DATA_BLOCK "MGUD"
TITLE =
VERSION : 0.1


  STRUCT
   ALB_BUFFER : INT ;
   VASS_BUFFER : INT ;
   ALB_GREZZI : INT ;
   VASS_GREZZI : INT ;
   ALB_FINITI : INT ;
   VASS_FINITI : INT ;
   ORIG_ALB_PP : INT ;
   ORIG_ALB_BSX_P1 : INT ;
   ORIG_ALB_BSX_P2 : INT ;
   ORIG_ALB_BDX_P1 : INT ;
   ORIG_ALB_BDX_P2 : INT ;
   ZN_CEN_PRE_BSX : INT ;
   ZN_CEN_OCC_BSX : INT ;
   ZN_CEN_PRE_BDX : INT ;
   ZN_CEN_OCC_BDX : INT ;
   ALB_ESTRATTI : INT ;
   VAR_DISP : INT ;
   VAR_DISP1 : INT ;
   VAR_DISP2 : INT ;
   VAR_DISP3 : INT ;
   VAR_DISP4 : INT ;
   VAR_DISP5 : INT ;
   VAR_DISP6 : INT ;
   VAR_DISP7 : INT ;
   VAR_DISP8 : INT ;
      Y_SX_ATTESA_MSX : REAL ;
   Y_SX_DISCESA_MSX : REAL ;
   Z_SX_ALTO : REAL ;
   Z_SX_PREL_MSX : REAL ;
   Z_SX_DEP_MSX : REAL ;
   Z_SX_SVINC_MSX : REAL ;
   C_SX_PREL_MSX : REAL ;
   A_SX_PREL_MSX : REAL ;
   A_SX_DEP_MSX : REAL ;
   MSX_DISP1 : REAL ;
   MSX_DISP2 : REAL ;
   MSX_DISP3 : REAL ;
   MSX_DISP4 : REAL ;
   MSX_DISP5 : REAL ;
   MSX_DISP6 : REAL ;
   MSX_DISP7 : REAL ;
   MSX_DISP8 : REAL ;
   Y_SX_DISCESA_PP : REAL ;
   Z_SX_ALTO_PP : REAL ;
   Z_SX_PREL_PP : REAL ;
   Z_SX_SVINC_PP : REAL ;
   C_SX_PREL_PP : REAL ;
   A_SX_PREL_PP : REAL ;
   A_SX_DEP_PP : REAL ;
   PP_DISP1 : REAL ;
   PP_DISP2 : REAL ;
   PP_DISP3 : REAL ;
   PP_DISP4 : REAL ;
   PP_DISP5 : REAL ;
   PP_DISP6 : REAL ;
   PP_DISP7 : REAL ;
   PP_DISP8 : REAL ;
   Z_SX_SVINC_PALLET : REAL ;
   Z_SX_PREL_PALLET : REAL ;
   Z_SX_DEP_PALLET : REAL ;
   Z_SX_PREL_ALBERI : REAL ;
   Y_SX_PREL_PALLET : REAL ;
   Y_SX_DEP_PALLET : REAL ;
   Y_SX_PREL_ALBERI : REAL ;
   A_SX_PREL_GREZZI : REAL ;
   C_SX_PREL_GREZZI : REAL ;
   A_SX_PREL_PALLET : REAL ;
   C_SX_PREL_PALLET : REAL ;
   Z_SX_DEP_ALBERI : REAL ;
   Y_SX_DEP_ALBERI : REAL ;
   A_SX_DEP_FINITI : REAL ;
   C_SX_DEP_FINITI : REAL ;
   DISP1 : REAL ;
   DISP2 : REAL ;
   DISP3 : REAL ;
   DISP4 : REAL ;
   DISP5 : REAL ;
   DISP6 : REAL ;
   DISP7 : REAL ;
   DISP8 : REAL ;
   DISP9 : REAL ;
   DISP10 : REAL ;
   DISP11 : REAL ;
   DISP12 : REAL ;
   DISP13 : REAL ;
   DISP14 : REAL ;
   DISP15 : REAL ;
   DISP16 : REAL ;
   Z_SX_PREL_PALLET_BUFF : REAL ;
   Z_SX_DEP_PALLET_BUFF : REAL ;
   Z_SX_PREL_ALBERI_BUFF : REAL ;
   Y_SX_PREL_ALBERI_BUFF_1 : REAL ;
   Y_SX_PREL_ALBERI_BUFF_2 : REAL ;
   Y_SX_DEP_PALLET_BUFF : REAL ;
   Z_SX_DEP_ONLINE : REAL ;
   Y_SX_DEP_ONLINE : REAL ;
   A_SX_DEP_ONLINE : REAL ;
   C_SX_DEP_ONLINE : REAL ;
   DISP18 : REAL ;
   DISP19 : REAL ;
   DISP20 : REAL ;
   DISP21 : REAL ;
   DISP22 : REAL ;
   DISP23 : REAL ;
   DISP24 : REAL ;
   DISP25 : REAL ;
   DISP26 : REAL ;
   DISP27 : REAL ;
   DISP28 : REAL ;
   DISP29 : REAL ;
   Y_SX_ATTESA_MDX : REAL ;
   Y_SX_DISCESA_MDX : REAL ;
   Z_SX_PREL_MDX : REAL ;
   Z_SX_DEP_MDX : REAL ;
   Z_SX_SVINC_MDX : REAL ;
   C_SX_PREL_MDX : REAL ;
   A_SX_PREL_MDX : REAL ;
   C_SX_DEP_MDX : REAL ;
   A_SX_DEP_MDX : REAL ;
   MDX_DISP1 : REAL ;
   MDX_DISP2 : REAL ;
   MDX_DISP3 : REAL ;
   MDX_DISP4 : REAL ;
   MDX_DISP5 : REAL ;
   MDX_DISP6 : REAL ;
   MDX_DISP7 : REAL ;
   MDX_DISP8 : REAL ;
   Y_DX_ATTESA_MSX : REAL ;
   Y_DX_DISCESA_MSX : REAL ;
   Z_DX_ALTO : REAL ;
   Z_DX_PREL_MSX : REAL ;
   Z_DX_DEP_MSX : REAL ;
   Z_DX_SVINC_MSX : REAL ;
   C_DX_PREL_MSX : REAL ;
   A_DX_PREL_MSX : REAL ;
   A_DX_DEP_MSX : REAL ;
   MSX_DISP9 : REAL ;
   MSX_DISP10 : REAL ;
   MSX_DISP11 : REAL ;
   MSX_DISP12 : REAL ;
   MSX_DISP13 : REAL ;
   MSX_DISP14 : REAL ;
   MSX_DISP15 : REAL ;
   MSX_DISP16 : REAL ;
   Y_DX_DISCESA_PP : REAL ;
   Z_DX_ALTO_PP : REAL ;
   Z_DX_PREL_PP : REAL ;
   Z_DX_SVINC_PP : REAL ;
   C_DX_PREL_PP : REAL ;
   A_DX_PREL_PP : REAL ;
   A_DX_DEP_PP : REAL ;
   PP_DISP9 : REAL ;
   PP_DISP10 : REAL ;
   PP_DISP11 : REAL ;
   PP_DISP12 : REAL ;
   PP_DISP13 : REAL ;
   PP_DISP14 : REAL ;
   PP_DISP15 : REAL ;
   PP_DISP16 : REAL ;
   Z_DX_SVINC_PALLET : REAL ;
   Z_DX_PREL_PALLET : REAL ;
   Z_DX_DEP_PALLET : REAL ;
   Z_DX_PREL_ALBERI : REAL ;
   Y_DX_PREL_PALLET : REAL ;
   Y_DX_DEP_PALLET : REAL ;
   Y_DX_PREL_ALBERI : REAL ;
   A_DX_PREL_GREZZI : REAL ;
   C_DX_PREL_GREZZI : REAL ;
   A_DX_PREL_PALLET : REAL ;
   C_DX_PREL_PALLET : REAL ;
   Z_DX_DEP_ALBERI : REAL ;
   Y_DX_DEP_ALBERI : REAL ;
   A_DX_DEP_FINITI : REAL ;
   C_DX_DEP_FINITI : REAL ;
   DISP30 : REAL ;
   DISP31 : REAL ;
   DISP32 : REAL ;
   DISP33 : REAL ;
   DISP34 : REAL ;
   DISP35 : REAL ;
   DISP36 : REAL ;
   DISP37 : REAL ;
   DISP38 : REAL ;
   DISP39 : REAL ;
   DISP40 : REAL ;
   DISP41 : REAL ;
   DISP42 : REAL ;
   DISP43 : REAL ;
   DISP44 : REAL ;
   DISP45 : REAL ;
   Z_DX_PREL_PALLET_BUFF : REAL ;
   Z_DX_DEP_PALLET_BUFF : REAL ;
   Z_DX_PREL_ALBERI_BUFF : REAL ;
   Y_DX_PREL_ALBERI_BUFF_1 : REAL ;
   Y_DX_PREL_ALBERI_BUFF_2 : REAL ;
   Y_DX_DEP_PALLET_BUFF : REAL ;
   Z_DX_DEP_ONLINE : REAL ;
   Y_DX_DEP_ONLINE : REAL ;
   A_DX_DEP_ONLINE : REAL ;
   C_DX_DEP_ONLINE : REAL ;
   DISP46 : REAL ;
   DISP47 : REAL ;
   DISP48 : REAL ;
   DISP49 : REAL ;
   DISP50 : REAL ;
   DISP51 : REAL ;
   DISP52 : REAL ;
   DISP53 : REAL ;
   DISP54 : REAL ;
   DISP55 : REAL ;
   DISP56 : REAL ;
   DISP57 : REAL ;
   Y_DX_ATTESA_MDX : REAL ;
   Y_DX_DISCESA_MDX : REAL ;
   Z_DX_PREL_MDX : REAL ;
   Z_DX_DEP_MDX : REAL ;
   Z_DX_SVINC_MDX : REAL ;
   C_DX_PREL_MDX : REAL ;
   A_DX_PREL_MDX : REAL ;
   C_DX_DEP_MDX : REAL ;
   A_DX_DEP_MDX : REAL ;
   MDX_DISP9 : REAL ;
   MDX_DISP10 : REAL ;
   MDX_DISP11 : REAL ;
   MDX_DISP12 : REAL ;
   MDX_DISP13 : REAL ;
   MDX_DISP14 : REAL ;
   MDX_DISP15 : REAL ;
   MDX_DISP16 : REAL ;
  END_STRUCT ;
BEGIN
   ALB_BUFFER := 0;
   VASS_BUFFER := 0;
   ALB_GREZZI := 0;
   VASS_GREZZI := 0;
   ALB_FINITI := 0;
   VASS_FINITI := 0;
   ORIG_ALB_PP := 0;
   ORIG_ALB_BSX_P1 := 0;
   ORIG_ALB_BSX_P2 := 0;
   ORIG_ALB_BDX_P1 := 0;
   ORIG_ALB_BDX_P2 := 0;
   ZN_CEN_PRE_BSX := 0;
   ZN_CEN_OCC_BSX := 0;
   ZN_CEN_PRE_BDX := 0;
   ZN_CEN_OCC_BDX := 0;
   ALB_ESTRATTI := 0;
   VAR_DISP := 0;
   VAR_DISP1 := 0;
   VAR_DISP2 := 0;
   VAR_DISP3 := 0;
   VAR_DISP4 := 0;
   VAR_DISP5 := 0;
   VAR_DISP6 := 0;
   VAR_DISP7 := 0;
   VAR_DISP8 := 0;
      Y_SX_ATTESA_MSX := 0.000000e+000 ;
   Y_SX_DISCESA_MSX := 0.000000e+000 ;
   Z_SX_ALTO := 0.000000e+000 ;
   Z_SX_PREL_MSX := 0.000000e+000 ;
   Z_SX_DEP_MSX := 0.000000e+000 ;
   Z_SX_SVINC_MSX := 0.000000e+000 ;
   C_SX_PREL_MSX := 0.000000e+000 ;
   A_SX_PREL_MSX := 0.000000e+000 ;
   A_SX_DEP_MSX := 0.000000e+000 ;
   MSX_DISP1 := 0.000000e+000 ;
   MSX_DISP2 := 0.000000e+000 ;
   MSX_DISP3 := 0.000000e+000 ;
   MSX_DISP4 := 0.000000e+000 ;
   MSX_DISP5 := 0.000000e+000 ;
   MSX_DISP6 := 0.000000e+000 ;
   MSX_DISP7 := 0.000000e+000 ;
   MSX_DISP8 := 0.000000e+000 ;
   Y_SX_DISCESA_PP := 0.000000e+000 ;
   Z_SX_ALTO_PP := 0.000000e+000 ;
   Z_SX_PREL_PP := 0.000000e+000 ;
   Z_SX_SVINC_PP := 0.000000e+000 ;
   C_SX_PREL_PP := 0.000000e+000 ;
   A_SX_PREL_PP := 0.000000e+000 ;
   A_SX_DEP_PP := 0.000000e+000 ;
   PP_DISP1 := 0.000000e+000 ;
   PP_DISP2 := 0.000000e+000 ;
   PP_DISP3 := 0.000000e+000 ;
   PP_DISP4 := 0.000000e+000 ;
   PP_DISP5 := 0.000000e+000 ;
   PP_DISP6 := 0.000000e+000 ;
   PP_DISP7 := 0.000000e+000 ;
   PP_DISP8 := 0.000000e+000 ;
   Z_SX_SVINC_PALLET := 0.000000e+000 ;
   Z_SX_PREL_PALLET := 0.000000e+000 ;
   Z_SX_DEP_PALLET := 0.000000e+000 ;
   Z_SX_PREL_ALBERI := 0.000000e+000 ;
   Y_SX_PREL_PALLET := 0.000000e+000 ;
   Y_SX_DEP_PALLET := 0.000000e+000 ;
   Y_SX_PREL_ALBERI := 0.000000e+000 ;
   A_SX_PREL_GREZZI := 0.000000e+000 ;
   C_SX_PREL_GREZZI := 0.000000e+000 ;
   A_SX_PREL_PALLET := 0.000000e+000 ;
   C_SX_PREL_PALLET := 0.000000e+000 ;
   Z_SX_DEP_ALBERI := 0.000000e+000 ;
   Y_SX_DEP_ALBERI := 0.000000e+000 ;
   A_SX_DEP_FINITI := 0.000000e+000 ;
   C_SX_DEP_FINITI := 0.000000e+000 ;
   DISP1 := 0.000000e+000 ;
   DISP2 := 0.000000e+000 ;
   DISP3 := 0.000000e+000 ;
   DISP4 := 0.000000e+000 ;
   DISP5 := 0.000000e+000 ;
   DISP6 := 0.000000e+000 ;
   DISP7 := 0.000000e+000 ;
   DISP8 := 0.000000e+000 ;
   DISP9 := 0.000000e+000 ;
   DISP10 := 0.000000e+000 ;
   DISP11 := 0.000000e+000 ;
   DISP12 := 0.000000e+000 ;
   DISP13 := 0.000000e+000 ;
   DISP14 := 0.000000e+000 ;
   DISP15 := 0.000000e+000 ;
   DISP16 := 0.000000e+000 ;
   Z_SX_PREL_PALLET_BUFF := 0.000000e+000 ;
   Z_SX_DEP_PALLET_BUFF := 0.000000e+000 ;
   Z_SX_PREL_ALBERI_BUFF := 0.000000e+000 ;
   Y_SX_PREL_ALBERI_BUFF_1 := 0.000000e+000 ;
   Y_SX_PREL_ALBERI_BUFF_2 := 0.000000e+000 ;
   Y_SX_DEP_PALLET_BUFF := 0.000000e+000 ;
   Z_SX_DEP_ONLINE := 0.000000e+000 ;
   Y_SX_DEP_ONLINE := 0.000000e+000 ;
   A_SX_DEP_ONLINE := 0.000000e+000 ;
   C_SX_DEP_ONLINE := 0.000000e+000 ;
   DISP18 := 0.000000e+000 ;
   DISP19 := 0.000000e+000 ;
   DISP20 := 0.000000e+000 ;
   DISP21 := 0.000000e+000 ;
   DISP22 := 0.000000e+000 ;
   DISP23 := 0.000000e+000 ;
   DISP24 := 0.000000e+000 ;
   DISP25 := 0.000000e+000 ;
   DISP26 := 0.000000e+000 ;
   DISP27 := 0.000000e+000 ;
   DISP28 := 0.000000e+000 ;
   DISP29 := 0.000000e+000 ;
   Y_SX_ATTESA_MDX := 0.000000e+000 ;
   Y_SX_DISCESA_MDX := 0.000000e+000 ;
   Z_SX_PREL_MDX := 0.000000e+000 ;
   Z_SX_DEP_MDX := 0.000000e+000 ;
   Z_SX_SVINC_MDX := 0.000000e+000 ;
   C_SX_PREL_MDX := 0.000000e+000 ;
   A_SX_PREL_MDX := 0.000000e+000 ;
   C_SX_DEP_MDX := 0.000000e+000 ;
   A_SX_DEP_MDX := 0.000000e+000 ;
   MDX_DISP1 := 0.000000e+000 ;
   MDX_DISP2 := 0.000000e+000 ;
   MDX_DISP3 := 0.000000e+000 ;
   MDX_DISP4 := 0.000000e+000 ;
   MDX_DISP5 := 0.000000e+000 ;
   MDX_DISP6 := 0.000000e+000 ;
   MDX_DISP7 := 0.000000e+000 ;
   MDX_DISP8 := 0.000000e+000 ;
   Y_DX_ATTESA_MSX := 0.000000e+000 ;
   Y_DX_DISCESA_MSX := 0.000000e+000 ;
   Z_DX_ALTO := 0.000000e+000 ;
   Z_DX_PREL_MSX := 0.000000e+000 ;
   Z_DX_DEP_MSX := 0.000000e+000 ;
   Z_DX_SVINC_MSX := 0.000000e+000 ;
   C_DX_PREL_MSX := 0.000000e+000 ;
   A_DX_PREL_MSX := 0.000000e+000 ;
   A_DX_DEP_MSX := 0.000000e+000 ;
   MSX_DISP9 := 0.000000e+000 ;
   MSX_DISP10 := 0.000000e+000 ;
   MSX_DISP11 := 0.000000e+000 ;
   MSX_DISP12 := 0.000000e+000 ;
   MSX_DISP13 := 0.000000e+000 ;
   MSX_DISP14 := 0.000000e+000 ;
   MSX_DISP15 := 0.000000e+000 ;
   MSX_DISP16 := 0.000000e+000 ;
   Y_DX_DISCESA_PP := 0.000000e+000 ;
   Z_DX_ALTO_PP := 0.000000e+000 ;
   Z_DX_PREL_PP := 0.000000e+000 ;
   Z_DX_SVINC_PP := 0.000000e+000 ;
   C_DX_PREL_PP := 0.000000e+000 ;
   A_DX_PREL_PP := 0.000000e+000 ;
   A_DX_DEP_PP := 0.000000e+000 ;
   PP_DISP9 := 0.000000e+000 ;
   PP_DISP10 := 0.000000e+000 ;
   PP_DISP11 := 0.000000e+000 ;
   PP_DISP12 := 0.000000e+000 ;
   PP_DISP13 := 0.000000e+000 ;
   PP_DISP14 := 0.000000e+000 ;
   PP_DISP15 := 0.000000e+000 ;
   PP_DISP16 := 0.000000e+000 ;
   Z_DX_SVINC_PALLET := 0.000000e+000 ;
   Z_DX_PREL_PALLET := 0.000000e+000 ;
   Z_DX_DEP_PALLET := 0.000000e+000 ;
   Z_DX_PREL_ALBERI := 0.000000e+000 ;
   Y_DX_PREL_PALLET := 0.000000e+000 ;
   Y_DX_DEP_PALLET := 0.000000e+000 ;
   Y_DX_PREL_ALBERI := 0.000000e+000 ;
   A_DX_PREL_GREZZI := 0.000000e+000 ;
   C_DX_PREL_GREZZI := 0.000000e+000 ;
   A_DX_PREL_PALLET := 0.000000e+000 ;
   C_DX_PREL_PALLET := 0.000000e+000 ;
   Z_DX_DEP_ALBERI := 0.000000e+000 ;
   Y_DX_DEP_ALBERI := 0.000000e+000 ;
   A_DX_DEP_FINITI := 0.000000e+000 ;
   C_DX_DEP_FINITI := 0.000000e+000 ;
   DISP30 := 0.000000e+000 ;
   DISP31 := 0.000000e+000 ;
   DISP32 := 0.000000e+000 ;
   DISP33 := 0.000000e+000 ;
   DISP34 := 0.000000e+000 ;
   DISP35 := 0.000000e+000 ;
   DISP36 := 0.000000e+000 ;
   DISP37 := 0.000000e+000 ;
   DISP38 := 0.000000e+000 ;
   DISP39 := 0.000000e+000 ;
   DISP40 := 0.000000e+000 ;
   DISP41 := 0.000000e+000 ;
   DISP42 := 0.000000e+000 ;
   DISP43 := 0.000000e+000 ;
   DISP44 := 0.000000e+000 ;
   DISP45 := 0.000000e+000 ;
   Z_DX_PREL_PALLET_BUFF := 0.000000e+000 ;
   Z_DX_DEP_PALLET_BUFF := 0.000000e+000 ;
   Z_DX_PREL_ALBERI_BUFF := 0.000000e+000 ;
   Y_DX_PREL_ALBERI_BUFF_1 := 0.000000e+000 ;
   Y_DX_PREL_ALBERI_BUFF_2 := 0.000000e+000 ;
   Y_DX_DEP_PALLET_BUFF := 0.000000e+000 ;
   Z_DX_DEP_ONLINE := 0.000000e+000 ;
   Y_DX_DEP_ONLINE := 0.000000e+000 ;
   A_DX_DEP_ONLINE := 0.000000e+000 ;
   C_DX_DEP_ONLINE := 0.000000e+000 ;
   DISP46 := 0.000000e+000 ;
   DISP47 := 0.000000e+000 ;
   DISP48 := 0.000000e+000 ;
   DISP49 := 0.000000e+000 ;
   DISP50 := 0.000000e+000 ;
   DISP51 := 0.000000e+000 ;
   DISP52 := 0.000000e+000 ;
   DISP53 := 0.000000e+000 ;
   DISP54 := 0.000000e+000 ;
   DISP55 := 0.000000e+000 ;
   DISP56 := 0.000000e+000 ;
   DISP57 := 0.000000e+000 ;
   Y_DX_ATTESA_MDX := 0.000000e+000 ;
   Y_DX_DISCESA_MDX := 0.000000e+000 ;
   Z_DX_PREL_MDX := 0.000000e+000 ;
   Z_DX_DEP_MDX := 0.000000e+000 ;
   Z_DX_SVINC_MDX := 0.000000e+000 ;
   C_DX_PREL_MDX := 0.000000e+000 ;
   A_DX_PREL_MDX := 0.000000e+000 ;
   C_DX_DEP_MDX := 0.000000e+000 ;
   A_DX_DEP_MDX := 0.000000e+000 ;
   MDX_DISP9 := 0.000000e+000 ;
   MDX_DISP10 := 0.000000e+000 ;
   MDX_DISP11 := 0.000000e+000 ;
   MDX_DISP12 := 0.000000e+000 ;
   MDX_DISP13 := 0.000000e+000 ;
   MDX_DISP14 := 0.000000e+000 ;
   MDX_DISP15 := 0.000000e+000 ;
   MDX_DISP16 := 0.000000e+000 ;

   END_DATA_BLOCK

